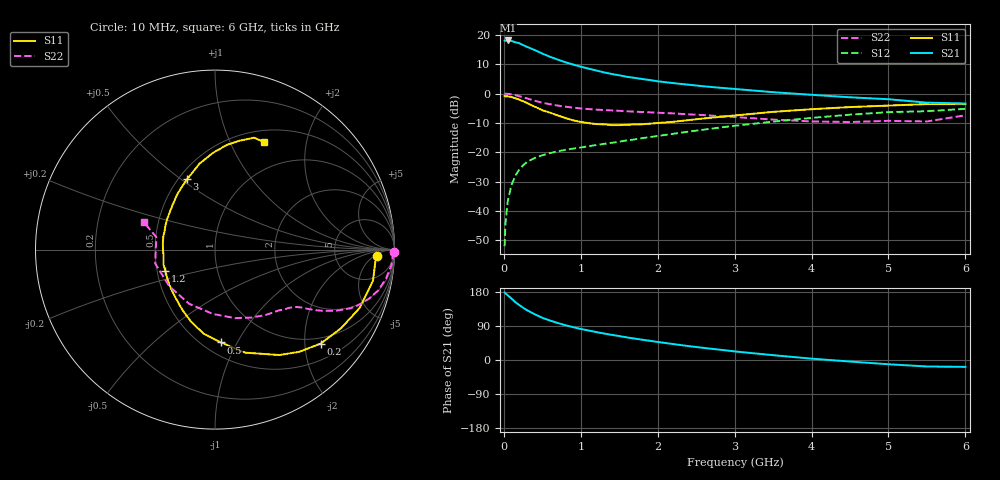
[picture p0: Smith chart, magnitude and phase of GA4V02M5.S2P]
! Infineon Technologies  Discrete & RF Semiconductors
! BF775
! Si NPN RF Bipolar Junction Transistor in SOT23
! VCE = 4 V  IC = 2.5 mA
! Common Emitter S-Parameters:  May  1996
# GHz  S  MA  R  50
!  f  S11  S21  S12  S22
! GHz  MAG  ANG  MAG  ANG  MAG  ANG  MAG  ANG
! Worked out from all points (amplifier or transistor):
!   36 points, 10 MHz to 6 GHz, reference 50 ohm
!   highest |S21| = 18.1 dB at 50 MHz (marker M1)
!   |S21| within 3 dB of that: start of sweep to 377.2 MHz
!   unconditionally stable (mu >= 1): 1.083 GHz to 3.547 GHz
!   at 250 MHz: K = 0.32, MSG = 20.5 dB, |S12| = -24.5 dB
!   at 1.4 GHz: K = 1.11, MAG = 9.7 dB, |S12| = -16.8 dB
!   at 6 GHz: K = 0.98, MSG = 0.9 dB, |S12| = -5.2 dB
!   S11 on the Smith chart (normalised r, x): 10 MHz: 17, -7; 200 MHz: 0.86, -2.37; 500 MHz: 0.61, -0.86; 1.2 GHz: 0.55, -0.15; 3 GHz: 0.55, +0.53; 6 GHz: 0.63, +1.35
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0.01  0.9053 -2.3  8.006 178.3  0.0025 87.6  0.9972 -0.9
0.02  0.8957 -4.3  7.882 176.2  0.0058 88.7  0.9916 -1.9
0.05  0.8972 -11.0  8.019 170.8  0.0144 83.9  0.9871 -5.0
0.1  0.8695 -21.9  7.846 162.0  0.0279 77.5  0.9659 -9.7
0.15  0.8279 -31.9  7.478 152.7  0.0398 71.9  0.9377 -14.0
0.2  0.7882 -41.6  7.19 145.1  0.0504 67.3  0.9006 -17.7
0.25  0.7379 -50.5  6.684 137.9  0.0596 63.1  0.8596 -20.9
0.3  0.689 -58.5  6.244 131.5  0.0681 60.3  0.8249 -23.3
0.4  0.5982 -73.7  5.52 120.9  0.0796 54.9  0.7545 -26.9
0.5  0.5185 -86.3  4.789 111.3  0.0885 51.7  0.6957 -29.4
0.6  0.472 -97.8  4.226 104.2  0.0966 49.7  0.656 -31.0
0.8  0.3817 -118.5  3.413 91.8  0.1097 47.5  0.5972 -33.2
0.9  0.3492 -128.4  3.116 86.6  0.1151 48.0  0.5737 -34.1
1.1  0.3128 -147.6  2.658 77.8  0.1263 48.2  0.5428 -36.3
1.2  0.3012 -156.4  2.466 73.8  0.1321 48.5  0.5315 -37.4
1.6  0.2927 173.2  1.927 59.6  0.1586 49.4  0.4982 -42.5
2.2  0.3288 139.7  1.505 42.1  0.2054 49.8  0.4583 -53.1
3  0.4217 111.6  1.196 22.7  0.2814 45.7  0.398 -73.7
3.5  0.4867 100.2  1.053 12.7  0.3315 41.1  0.3588 -91.8
4.5  0.5872 83.5  0.862 -4.1  0.4358 28.8  0.3264 -141.4
5.5  0.6602 70.8  0.698 -17.1  0.4993 13.1  0.3338 168.1
6  0.6588 65.7  0.676 -18.2  0.5482 8.7  0.4253 158.9
